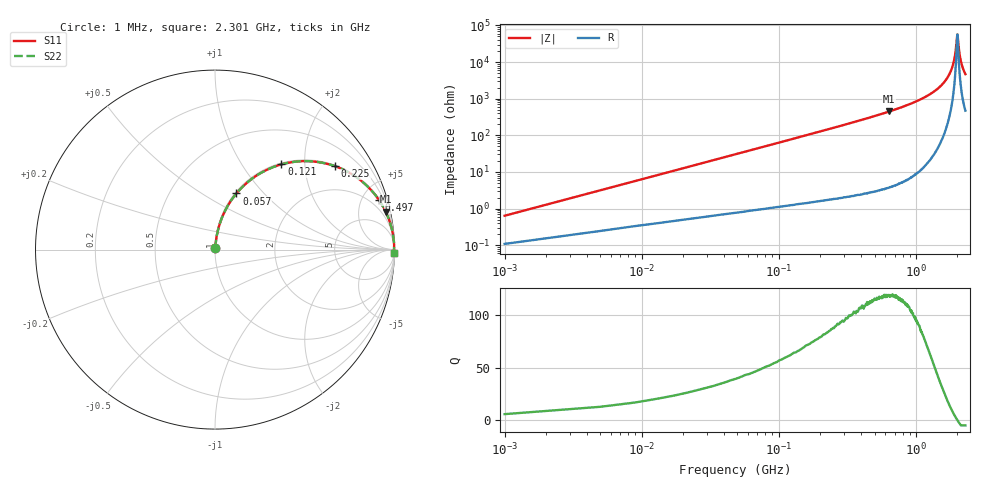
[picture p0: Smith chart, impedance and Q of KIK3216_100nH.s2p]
!version-2
!date-01.2022
!Series
# MHz S RI R 50
!Freq ReS11 ImS11 ReS21 ImS21 ReS12 ImS12 ReS22 ImS22
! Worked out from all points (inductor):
!   576 points, 1 MHz to 2.301 GHz, reference 50 ohm
!   read as one part in series: L = 100 nH near 9 MHz
!   highest Q = 119 at 641 MHz (marker M1), where L = 111 nH
!   self-resonance near 2.009 GHz
!   S11 on the Smith chart (normalised r, x): 1 MHz: 1.00, +0.01; 57 MHz: 1.02, +0.72; 121 MHz: 1.02, +1.53; 225 MHz: 1.03, +2.86; 497 MHz: 1.06, +6.65; 2.301 GHz: 10, -93
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1  0.00114 0.00627  0.9989 -0.00627  0.9989 -0.00627  0.00114 0.00627
13  0.0105 0.0805  0.9895 -0.0805  0.9895 -0.0805  0.0105 0.0805
21  0.0219 0.1284  0.9781 -0.1284  0.9781 -0.1284  0.0219 0.1284
37  0.057 0.2178  0.943 -0.2178  0.943 -0.2178  0.057 0.2178
57  0.1195 0.313  0.8805 -0.313  0.8805 -0.313  0.1195 0.313
121  0.37 0.4748  0.63 -0.4748  0.63 -0.4748  0.37 0.4748
225  0.6702 0.4642  0.3298 -0.4642  0.3298 -0.4642  0.6702 0.4642
385  0.8608 0.3415  0.1392 -0.3415  0.1392 -0.3415  0.8608 0.3415
497  0.9151 0.2744  0.0849 -0.2744  0.0849 -0.2744  0.9151 0.2744
641  0.951 0.2117  0.049 -0.2117  0.049 -0.2117  0.951 0.2117
769  0.9683 0.1708  0.0317 -0.1708  0.0317 -0.1708  0.9683 0.1708
1153  0.9903 0.0917  0.00968 -0.0917  0.00968 -0.0917  0.9903 0.0917
1537  0.9968 0.0429  0.00316 -0.0429  0.00316 -0.0429  0.9968 0.0429
1781  0.9981 0.0192  0.00188 -0.0192  0.00188 -0.0192  0.9981 0.0192
1921  0.9983 0.00728  0.0017 -0.00728  0.0017 -0.00728  0.9983 0.00728
1961  0.9983 0.00402  0.00171 -0.00402  0.00171 -0.00402  0.9983 0.00402
2001  0.9983 0.000841  0.00174 -0.000841  0.00174 -0.000841  0.9983 0.000841
2013  0.9982 -0.000101  0.00176 0.000101  0.00176 0.000101  0.9982 -0.000101
2073  0.9981 -0.00473  0.00185 0.00473  0.00185 0.00473  0.9981 -0.00473
2121  0.998 -0.00834  0.00196 0.00834  0.00196 0.00834  0.998 -0.00834
2201  0.9978 -0.0142  0.0022 0.0142  0.0022 0.0142  0.9978 -0.0142
2301  0.9974 -0.0211  0.00259 0.0211  0.00259 0.0211  0.9974 -0.0211
